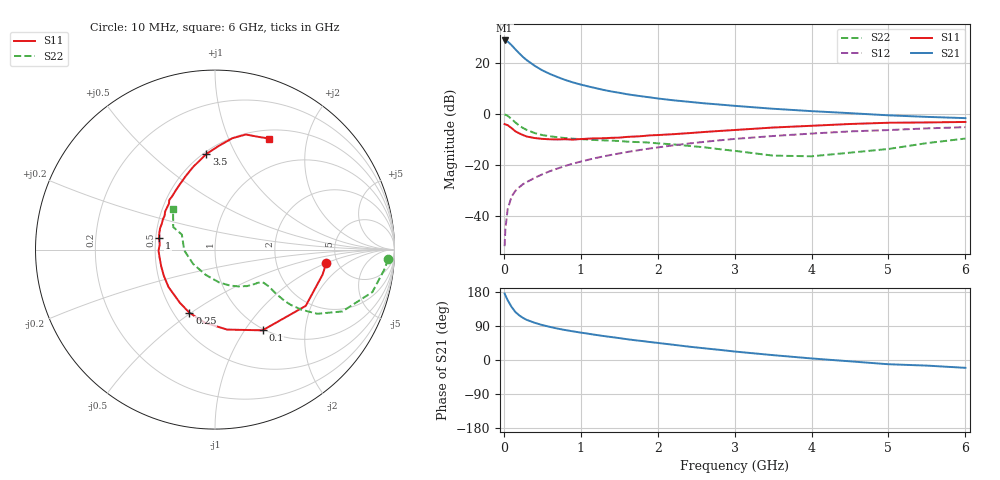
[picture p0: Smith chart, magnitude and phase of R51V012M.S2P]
! SIEMENS Small Signal Semiconductors
! BFR183
! Si NPN RF Bipolar Junction Transistor in SOT23
! VCE = 1 V  IC = 12 mA
! Common Emitter S-Parameters:  May  1996
# GHz  S  MA  R  50
!  f  S11  S21  S12  S22
! GHz  MAG  ANG  MAG  ANG  MAG  ANG  MAG  ANG
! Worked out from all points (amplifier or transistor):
!   36 points, 10 MHz to 6 GHz, reference 50 ohm
!   highest |S21| = 28.8 dB at 10 MHz (marker M1)
!   |S21| within 3 dB of that: start of sweep to 135.4 MHz
!   unconditionally stable (mu >= 1): 638 MHz to 2.68 GHz
!   at 250 MHz: K = 0.70, MSG = 25.0 dB, |S12| = -27.7 dB
!   at 1.4 GHz: K = 1.07, MAG = 10.8 dB, |S12| = -16.2 dB
!   at 6 GHz: K = 0.93, MSG = 1.8 dB, |S12| = -5.3 dB
!   S11 on the Smith chart (normalised r, x): 10 MHz: 4.08, -0.99; 100 MHz: 0.98, -1.21; 250 MHz: 0.60, -0.49; 1 GHz: 0.52, +0.07; 3.5 GHz: 0.52, +0.77; 6 GHz: 0.61, +1.42
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0.01  0.6251 -6.8  27.44 175.4  0.0025 87.9  0.9656 -3.1
0.02  0.6151 -13.2  27.38 170.6  0.0054 84.8  0.9525 -6.3
0.05  0.5948 -31.8  26.09 157.8  0.0134 76.9  0.9082 -15.1
0.1  0.522 -59.5  22.21 140.3  0.0234 66.9  0.7888 -25.9
0.15  0.4507 -81.4  18.38 126.7  0.0305 62.8  0.6728 -32.1
0.2  0.4111 -98.0  15.34 117.9  0.0359 61.7  0.5866 -34.8
0.25  0.3796 -112.1  12.97 110.9  0.0414 60.7  0.5231 -36.1
0.3  0.3549 -123.5  11.2 105.7  0.0456 61.4  0.4782 -36.4
0.4  0.3326 -141.1  8.75 98.3  0.0549 62.6  0.4166 -35.8
0.5  0.3203 -152.9  7.108 92.2  0.0645 63.9  0.3806 -34.9
0.6  0.314 -162.3  6.026 87.3  0.0744 64.5  0.36 -34.4
0.7  0.312 -171.7  5.225 82.8  0.084 65.1  0.3447 -34.3
0.8  0.3146 -179.1  4.588 79.0  0.0943 64.8  0.332 -34.3
1  0.3175 168.5  3.732 72.3  0.1145 64.7  0.3165 -35.2
1.1  0.3237 163.4  3.425 69.3  0.1247 64.4  0.3109 -36.5
1.3  0.3296 154.1  2.923 63.2  0.1456 62.9  0.2993 -38.5
1.6  0.3499 142.5  2.415 54.9  0.1765 60.4  0.283 -43.2
2.2  0.3956 123.6  1.835 40.3  0.2386 54.3  0.2498 -55.6
3.5  0.5348 95.2  1.25 12.8  0.3644 37.4  0.1501 -110.0
4.5  0.6276 81.2  1.024 -3.5  0.4487 24.2  0.1715 -178.6
5.5  0.6732 68.9  0.866 -14.8  0.5147 12.4  0.2644 151.7
6  0.6881 64.0  0.818 -20.7  0.5442 4.8  0.3247 136.0
